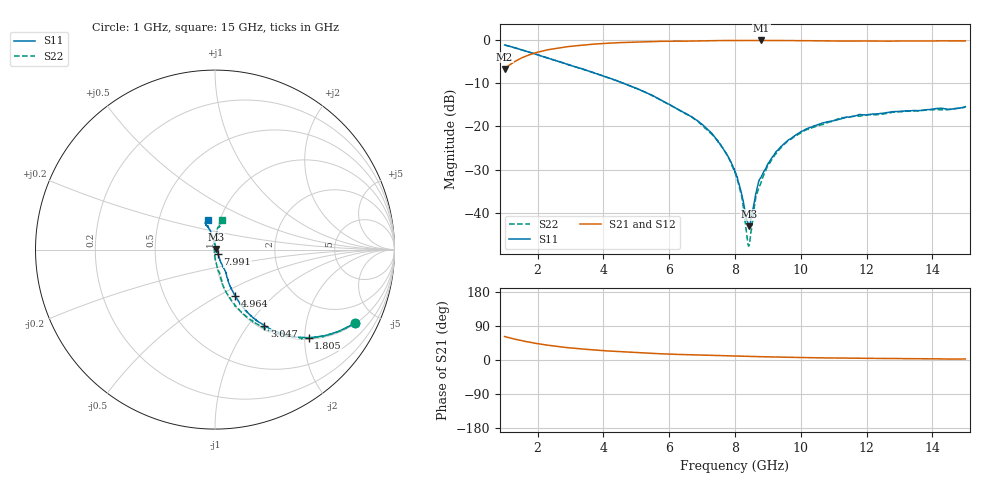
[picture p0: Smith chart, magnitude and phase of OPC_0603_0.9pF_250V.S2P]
! FILE NAME
! DATE 08/21/2012  13:50
! CORRECTED  DATA
# GHz  S  MA  R  50.00
!  FREQ  S11M  S11A  S21M  S21A  S12M  S12A  S22M  S22A
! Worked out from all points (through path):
!   1601 points, 1 GHz to 15 GHz, reference 50 ohm
!   highest |S21| = -0.06 dB at 8.796 GHz (marker M1); lowest = -6.7 dB at 1 GHz (marker M2)
!   lowest |S11| = -43.2 dB at 8.429 GHz (marker M3), VSWR 1.01, Z = 50.6 + j0.301 ohm
!   |S11| at or under -10 dB: 4.61 GHz to end of sweep
!   |S22| runs from -47.8 to -1.1 dB; largest |S21 - S12| = 0.0082
!   S11 on the Smith chart (normalised r, x): 1 GHz: 1.06, -3.79; 1.805 GHz: 1.04, -2.09; 3.047 GHz: 1.06, -1.20; 4.964 GHz: 1.07, -0.60; 7.991 GHz: 1.03, -0.05; 15 GHz: 0.87, +0.30
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1  0.8788 -27.7  0.4639 61.9  0.4638 61.8  0.8787 -27.7
1.805  0.7155 -43.2  0.6876 46.2  0.6876 46.2  0.7155 -43.5
3.0475  0.505 -56.9  0.8519 31.4  0.8513 31.5  0.5045 -58.7
3.33625  0.4672 -59.1  0.8748 29.2  0.8743 29.2  0.4658 -61.3
4.96375  0.281 -66.7  0.9526 19.7  0.9527 19.7  0.2781 -73.3
5.6725  0.2101 -67.6  0.9692 16.7  0.9691 16.7  0.2092 -77.2
7.23  0.08792 -64.7  0.9864 12.4  0.9864 12.4  0.08514 -83.5
7.67625  0.05246 -62.2  0.9901 11.2  0.9897 11.2  0.05257 -88.9
7.99125  0.03004 -57.6  0.9918 10.4  0.991 10.4  0.03007 -93.8
8  0.02984 -56.3  0.9917 10.4  0.991 10.4  0.0292 -95.3
8.175  0.01839 -47.9  0.9914 9.9  0.9916 10.0  0.01687 -99.8
8.3675  0.008026 -5.1  0.991 9.6  0.9909 9.6  0.005076 -139.3
8.42875  0.006916 25.4  0.9916 9.5  0.9912 9.5  0.004157 167.0
8.48125  0.008404 53.3  0.9913 9.3  0.9909 9.4  0.005766 131.1
8.6475  0.01746 84.0  0.9909 9.0  0.991 9.0  0.01575 99.6
8.79625  0.02587 87.7  0.9927 8.7  0.9919 8.7  0.02267 96.7
9.0325  0.0382 96.2  0.9907 8.2  0.9906 8.3  0.03645 93.3
9.40875  0.05896 100.1  0.99 7.6  0.9894 7.6  0.05723 90.9
10.33625  0.09882 103.2  0.9854 6.1  0.9847 6.1  0.09605 83.7
11.2375  0.1229 106.5  0.9768 5.1  0.9767 5.2  0.1263 81.3
12.6725  0.1457 110.2  0.9738 4.0  0.9739 4.0  0.1428 79.4
15  0.1695 104.1  0.9813 2.8  0.981 2.8  0.1673 77.1
